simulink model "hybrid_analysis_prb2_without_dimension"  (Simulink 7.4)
settings: Solver=ode4  SolverMode=SingleTasking  StartTime=0.0  StopTime=60.0  FixedStep=0.0005  RelTol=1e-3
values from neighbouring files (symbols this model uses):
  AR1 = 1    [prb2.m]
  AR2 = 4.125    [prb2.m]
  AR3 = 1    [prb2.m]
  c1_mu1 = 1    [prb2.m]
  c1_mu2 = 1    [prb2.m]
  c2_mu1 = 0.1316    [prb2.m]
  c2_mu2 = 0.0001748    [prb2.m]
  c3_mu1 = 1    [prb2.m]
  c3_mu2 = 1    [prb2.m]
  Hf = 0.310    (= 0.31)    [prb2.m]
  Ici = 0.009020    (= 0.00902)    [prb2.m]
  Ici12 = It2 - It    (= 0.0149238079833)    [prb2.m]
  Icr = 0.005806    [prb2.m]
  Icr12 = Icr + Isi/(R1*R1) + Ici/(R2*R2)    (= 0.0366753653)    [prb2.m]
  Isi = 0.001020    (= 0.00102)    [prb2.m]
  Isi12 = It1 - It    (= 0.00429856082609)    [prb2.m]
  Isr = 1    [prb2.m]
  It = 0.05623    [prb2.m]
  It1 = It + Isi + R1*R1*Icr + R1*R1*Ici/(R2*R2)    (= 0.0605285608261)    [prb2.m]
  It2 = It + Ici + R2*R2*Icr + R2*R2*Isi/(R1*R1)    (= 0.0711538079833)    [prb2.m]
  Iwf = 2.8    [prb2.m]
  Ks = 6742.0    (= 6742)    [prb2.m]
  M = 1644.0 + 125.0    (= 1769)    [prb2.m]
  m_s_to_km_h = 3.6    [prb2.m]
  Pc1init = 0    [prb2.m]
  Pc1max = 1    [prb2.m]
  Pc2init = 0    [prb2.m]
  Pc2max = 400.0    (= 400)    [prb2.m]
  Pc3init = 0    [prb2.m]
  Pc3max = 1    [prb2.m]
  pres_index = [-5,5]    [prb2.m]
  R1 = Rci*Rsi/(1-Rci*Rcr)    (= 0.342353138929)    [prb2.m]
  R2 = Rci    (= 0.6379)    [prb2.m]
  R4 = 1    [prb2.m]
  Rci = 0.6379    [prb2.m]
  Rcr = 0.7045    [prb2.m]
  Rd = 0.3521    [prb2.m]
  Rr = 1    [prb2.m]
  Rsi = 0.2955    [prb2.m]
  Rsr = 1    [prb2.m]
  tau1off = 0    [prb2.m]
  tau1on = 1    [prb2.m]
  tau2off = 0    [prb2.m]
  tau2on = 1    [prb2.m]
  tau3off = 0    [prb2.m]
  tau3on = 1    [prb2.m]
  Ts_init = 0    [prb2.m]
  V_init = 0    [prb2.m]
  Wt_init = 0    [prb2.m]
undefined symbols (not defined in the file or in its folder): c1_table, c2_table, c3_table, shift_1_2, shift_2_1, trans, trans_v1_1
libraries: simulink x1
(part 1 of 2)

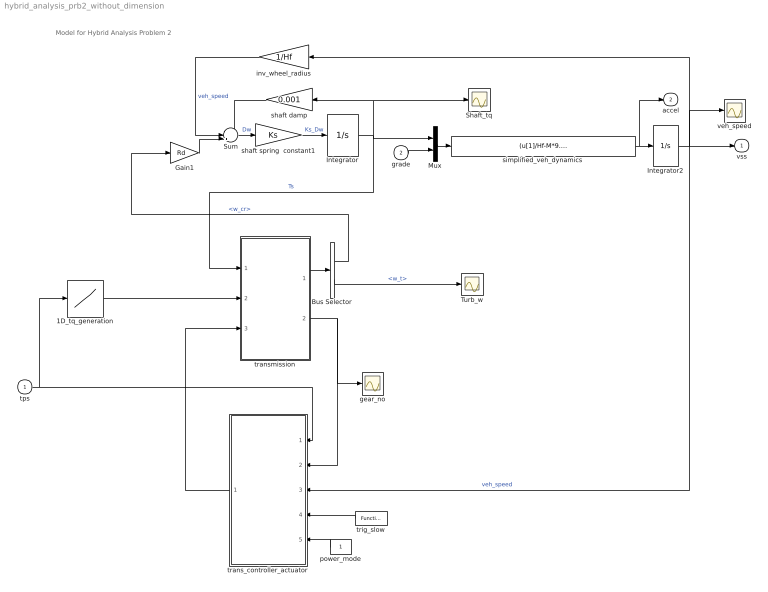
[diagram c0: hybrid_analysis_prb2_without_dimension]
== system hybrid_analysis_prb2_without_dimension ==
  note: Model for Hybrid Analysis Problem 2
  tps : Inport  Description=|
      | begin dimension       
      | output _ : [(scalar)];
      | end dimension
  grade : Inport  Description=|  Port=2
      | begin dimension               
      | output _ : [(angle radian 1)];
      | end dimension
  1D_tq_generation : Lookup  Description=|  InputValues=[0 100]  Table=[30 200]
      | begin dimension                                                
      | input 1 : [(scalar)];                                          
      | output 1 : [(length metre 2, mass kilogram 1, time second -2)];
      | end dimension
  Bus Selector : BusSelector  OutputSignals=w_cr,w_t
  Gain1 : Gain  Gain=Rd
  Integrator : Integrator  InitialCondition=Ts_init
  Integrator2 : Integrator  InitialCondition=V_init
  Mux : Mux  Inputs=2
  Shaft_tq : Scope
  Sum : Sum  Inputs=--+
  Turb_w : Scope
  gear_no : Scope
  inv_wheel_radius : Gain  Description=|  Gain=1/Hf
      | begin dimension                  
      | constant 1 : [(length metre -1)];
      | end dimension
  power_mode : Constant  Description=|
      | begin dimension       
      | output _ : [(scalar)];
      | end dimension
  shaft damp : Gain  Gain=0.001
  shaft spring  constant1 : Gain  Gain=Ks
  simplified_veh_dynamics : Fcn  Expr=(u[1]/Hf-M*9.81*sin(u[2]))/(M+2*Iwf/(Hf*Hf))
  trans_controller_actuator : Subsystem  AncestorBlock=trans/trans_v1_1
  transmission : Subsystem
  trig_slow : simulink/Ports & Subsystems/Function-Call Generator  sample_time=.001  numberOfIterations=1
  veh_speed : Scope
  vss : Outport  Description=|
      | begin dimension                              
      | input _ : [(length metre 1, time second -1)];
      | end dimension
  accel : Outport  Description=|  Port=2
      | begin dimension                              
      | input _ : [(length metre 1, time second -2)];
      | end dimension
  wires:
  transmission/2(current_gear) -> trans_controller_actuator/2(a_gear), gear_no/1
  power_mode/1 -> trans_controller_actuator/5(p_e_switch)
  simplified_veh_dynamics/1 -> Integrator2/1, accel/1
  Mux/1 -> simplified_veh_dynamics/1
  Integrator2/1 -> trans_controller_actuator/3(vss), vss/1, veh_speed/1, inv_wheel_radius/1  "veh_speed"
  grade/1 -> Mux/2
  transmission/1(omegas) -> Bus Selector/1
  tps/1 -> trans_controller_actuator/1(tps), 1D_tq_generation/1
  Integrator/1 -> Mux/1, Shaft_tq/1, shaft damp/1, transmission/1(T_s)  "Ts"
  trig_slow/1 -> trans_controller_actuator/4(trig_trans_slow)
  Sum/1 -> shaft spring  constant1/1  "Dw"
  shaft spring  constant1/1 -> Integrator/1  "Ks_Dw"
  Bus Selector/1 -> Gain1/1  "<w_cr>"
  inv_wheel_radius/1 -> Sum/2  "veh_speed"
  1D_tq_generation/1 -> transmission/2(T_t)
  trans_controller_actuator/1(pcs) -> transmission/3(pc)
  Gain1/1 -> Sum/3
  shaft damp/1 -> Sum/1
  Bus Selector/2 -> Turb_w/1  "<w_t>"

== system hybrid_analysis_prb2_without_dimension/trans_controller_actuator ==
  note: "Execution Context Diagram" At this level, 1 Simulink Subsystem per execution context (e.g. background, pip, cid, 1ms, 2ms, 4ms, etc.) is required. There are no C-specs at this level.
  tps : Inport
  a_gear : Inport  Port=2
  vss : Inport  Port=3
  trig_trans_slow : Inport  Port=4
  p_e_switch : Inport  Port=5
  IC : InitialCondition  Value=Pc1init
  IC1 : InitialCondition  Value=Pc2init
  IC2 : InitialCondition  Value=Pc3init
  Mux6 : Mux  Inputs=3
  Mux7 : Mux  Inputs=3
  clutch_actuators : Subsystem
  trans_slow : Subsystem
  pcs : Outport  InitialOutput=0
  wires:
  a_gear/1 -> trans_slow/5(a_gear)
  p_e_switch/1 -> trans_slow/4(p_e_switch)
  vss/1 -> trans_slow/3(vss)
  tps/1 -> trans_slow/2(tps)
  trig_trans_slow/1 -> trans_slow/1(trig_trans_slow)
  trans_slow/1(Pc1) -> IC/1
  trans_slow/2(Pc2) -> IC1/1
  IC/1 -> Mux7/1  "pc1"
  IC2/1 -> Mux7/3  "pc3"
  IC1/1 -> Mux7/2  "pc2"
  clutch_actuators/1(pc1) -> Mux6/1
  clutch_actuators/2(pc2) -> Mux6/2
  clutch_actuators/3(pc3) -> Mux6/3
  Mux6/1 -> pcs/1
  Mux7/1 -> clutch_actuators/1(pcs)
  trans_slow/3(Pc3) -> IC2/1

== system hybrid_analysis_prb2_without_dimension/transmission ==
  note: References: - Kim, J. and Cho, D., "An Automatic Transmission Model for Vehicle Control," Proc. IEEE Conf. on ITS, Nov. 1997, pp. 759-764. - D. Cho and J.K. Hedrick: "Automotive Powertrain Modeling for Control", ASME Trans. V111, Dec. 1989, pp. 568-576. - Butts, K., "Analysis Needs for Automotive Powertrain Control," Proceedings of The 7th Mechatronics Forum International Conference, September 6-8 2000, Atlanta, Georgia.
  T_s : Inport  Description=|
      | begin dimension                                                
      | output _ : [(length metre 2, mass kilogram 1, time second -2)];
      | end dimension
  T_t : Inport  Description=|  Port=2
      | begin dimension                                                
      | output _ : [(length metre 2, mass kilogram 1, time second -2)];
      | end dimension
  pc : Inport  Description=|  Port=3
      | begin dimension                                                 
      | output _ : [(length metre -1, mass kilogram 1, time second -2)];
      | end dimension
  Memory : Memory  X0=1
  Memory1 : Memory  X0=1
  compute_states : Subsystem
  pressure_to_torque : Subsystem
  reaction_torques : Subsystem
  omegas : Outport  Description=|
      | begin dimension                               
      | output _ : [(angle radian 1, time second -1)];
      | end dimension
  current_gear : Outport  Description=|  Port=2
      | begin dimension      
      | input _ : [(scalar)];
      | end dimension
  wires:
  pc/1 -> pressure_to_torque/1(pcs)
  T_t/1 -> reaction_torques/2(T_t), compute_states/2(T_t)
  T_s/1 -> reaction_torques/1(T_s), compute_states/1(T_s)
  pressure_to_torque/1(T_c) -> reaction_torques/3(T_c), compute_states/3(T_c)
  compute_states/3(gear) -> current_gear/1, Memory/1
  compute_states/1(states) -> omegas/1
  compute_states/2(derivatives) -> Memory1/1
  Memory1/1 -> reaction_torques/4(omega_dots)
  Memory/1 -> reaction_torques/5(current_gear)
  reaction_torques/1(RTs) -> compute_states/4(RTs)

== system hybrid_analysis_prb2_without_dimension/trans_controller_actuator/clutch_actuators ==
  note: This models the application of hydraulic pressure to the clutches and bands as first order lags Pc/Pc_max = 1/(tau*s +1) where each clutch has a distinct tau_on and tau_off.
  pcs : Inport
  Demux : Demux  Outputs=3
  Integrator : Integrator  InitialCondition=[Pc1init,Pc2init,Pc3init]
  Mux3 : Mux  Inputs=3
  Product2 : Product  Inputs=*/
  Sum3 : Sum  Inputs=-+|
  check_pc1 : Subsystem
  check_pc2 : Subsystem
  check_pc3 : Subsystem
  clutch_time_constant : Subsystem
  pc1 : Outport
  pc2 : Outport  Port=2
  pc3 : Outport  Port=3
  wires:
  Product2/1 -> Integrator/1
  Integrator/1 -> Demux/1, Sum3/1
  clutch_time_constant/3(tau3) -> Mux3/3
  clutch_time_constant/2(tau2) -> Mux3/2
  clutch_time_constant/1(tau1) -> Mux3/1
  Mux3/1 -> Product2/2
  pcs/1 -> Sum3/2, clutch_time_constant/1(pcs)
  Sum3/1 -> Product2/1
  check_pc1/1(pc1) -> pc1/1
  check_pc2/1(pc2) -> pc2/1
  check_pc3/1(pc3) -> pc3/1
  Demux/2 -> check_pc2/1(pcs)  "pc2"
  Demux/1 -> check_pc1/1(pcs)  "pc1"
  Demux/3 -> check_pc3/1(pcs)  "pc3"

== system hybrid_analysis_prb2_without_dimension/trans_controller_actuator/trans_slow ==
  note: Note: The controller should control clutch pressures and not torques. This will be fixed in the next release.
  trig_trans_slow : Inport
  tps : Inport  Port=2
  vss : Inport  Port=3
  p_e_switch : Inport  Port=4
  a_gear : Inport  Port=5
  trans_slow_ctl : Stateflow chart  TreatAsAtomicUnit=on
  trans_slow_torques : Subsystem  TreatAsAtomicUnit=on
  Pc1 : Outport  InitialOutput=0
  Pc2 : Outport  Port=2  InitialOutput=0
  Pc3 : Outport  Port=3  InitialOutput=0
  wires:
  trans_slow_torques/3(Pc3) -> Pc3/1
  trans_slow_torques/2(Pc2) -> Pc2/1
  trans_slow_torques/1(Pc1) -> Pc1/1
  trans_slow_ctl/1(do_trans_slow_torques) -> trans_slow_torques/Trigger  "do_trans_slow_torques"
  trig_trans_slow/1 -> trans_slow_ctl/Trigger
  a_gear/1 -> trans_slow_torques/4(a_gear)
  p_e_switch/1 -> trans_slow_torques/3(p_e_switch)
  vss/1 -> trans_slow_torques/2(vss)
  tps/1 -> trans_slow_torques/1(tps)

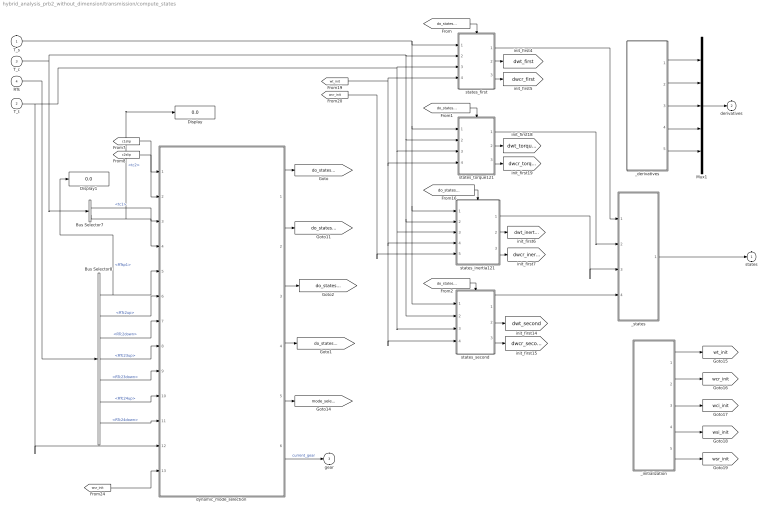
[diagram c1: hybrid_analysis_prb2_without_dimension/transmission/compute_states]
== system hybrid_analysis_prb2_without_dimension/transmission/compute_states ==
  T_s : Inport
  T_t : Inport  Port=2
  T_c : Inport  Port=3
  RTs : Inport  Port=4
  Bus Selector7 : BusSelector  OutputSignals=tc1,tc2
  Bus Selector8 : BusSelector  OutputSignals=RTsp1,RTc2up,RTc2down,RTc23up,RTc23down,RTc24up,RTc24down
  Display : Display
  Display1 : Display
  Mux1 : Mux  Inputs=5
  _derivatives : Subsystem  Description=Merge
  _initialization : Subsystem  Description=Merge
  _states : Subsystem  Description=Merge
  dynamic_mode_selection : Stateflow chart
  states_first : Subsystem  TreatAsAtomicUnit=on
  states_inertia121 : Subsystem  TreatAsAtomicUnit=on
  states_second : Subsystem  TreatAsAtomicUnit=on
  states_torque121 : Subsystem  TreatAsAtomicUnit=on
  states : Outport
  derivatives : Outport  Port=2
  gear : Outport  Port=3
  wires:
  [do_states_second] -> states_second/Enable
  [do_states_inertia121] -> states_inertia121/Enable
  [do_states_torque121] -> states_torque121/Enable
  [c2slip] -> dynamic_mode_selection/2(c2slip)
  [c1slip] -> dynamic_mode_selection/1(c1slip)
  Bus Selector7/1 -> dynamic_mode_selection/3(Tc1)  "<tc1>"
  T_c/1 -> Bus Selector7/1, states_first/2(T_c), states_torque121/2(T_c), states_inertia121/2(T_c), states_second/2(T_c)
  T_t/1 -> dynamic_mode_selection/12(Tt), states_first/3(T_t), states_torque121/3(T_t), states_inertia121/3(T_t), states_second/3(T_t)
  [do_states_first] -> states_first/Enable
  T_s/1 -> states_first/1(T_s), states_torque121/1(T_s), states_inertia121/1(T_s), states_second/1(T_s)
  states_first/1(states) -> _states/1(omegas)
  states_torque121/1(states) -> _states/2(omegas1)
  states_inertia121/1(states) -> _states/3(omegas2)
  states_second/1(states) -> _states/4(omegas3)
  [wt_init] -> states_first/4(wt_init), states_torque121/4(wt_init), states_inertia121/4(wt_init), states_second/4(wt_init1)
  [wcr_init] -> states_inertia121/5(wcr_init)
  states_first/2(wt_dot) -> [dwt_first]
  states_first/3(wcr_dot) -> [dwcr_first]
  states_torque121/2(wt_dot) -> [dwt_torque121]
  states_torque121/3(wcr_dot) -> [dwcr_torque121]
  states_inertia121/2(wt_dot) -> [dwt_inertia121]
  states_inertia121/3(wcr_dot) -> [dwcr_inertia121]
  states_second/2(wt_dot) -> [dwt_second]
  states_second/3(wcr_dot) -> [dwcr_second]
  _initialization/5(wsr_init) -> [wsr_init]
  _initialization/4(wsi_init) -> [wsi_init]
  _states/1(reaction_torques) -> states/1
  _derivatives/1(wt_dot) -> Mux1/1
  _derivatives/2(wcr_dot) -> Mux1/2
  _derivatives/3(wci_dot) -> Mux1/3
  _derivatives/4(wsi_dot) -> Mux1/4
  _derivatives/5(wsr_dot) -> Mux1/5
  Mux1/1 -> derivatives/1
  _initialization/1(wt_init) -> [wt_init]
  _initialization/3(wci_init) -> [wci_init]
  _initialization/2(wcr_init) -> [wcr_init]
  Bus Selector7/2 -> dynamic_mode_selection/4(Tc2), Display/1  "<tc2>"
  dynamic_mode_selection/6(a_gear) -> gear/1  "current_gear"
  dynamic_mode_selection/4(second) -> [do_states_second]
  dynamic_mode_selection/1(first) -> [do_states_first]
  dynamic_mode_selection/5(mode_select) -> [mode_select]
  Bus Selector8/1 -> dynamic_mode_selection/5(RTsp1), Display1/1  "<RTsp1>"
  RTs/1 -> Bus Selector8/1
  Bus Selector8/3 -> dynamic_mode_selection/7(RTc2down)  "<RTc2down>"
  Bus Selector8/4 -> dynamic_mode_selection/8(RTc23up)  "<RTc23up>"
  Bus Selector8/5 -> dynamic_mode_selection/9(RTc23down)  "<RTc23down>"
  Bus Selector8/6 -> dynamic_mode_selection/10(RTc24up)  "<RTc24up>"
  Bus Selector8/7 -> dynamic_mode_selection/11(RTc24down)  "<RTc24down>"
  Bus Selector8/2 -> dynamic_mode_selection/6(RTc2up)  "<RTc2up>"
  [wsr_init] -> dynamic_mode_selection/13(w_sr)
  dynamic_mode_selection/2(torque121) -> [do_states_torque121]
  dynamic_mode_selection/3(inertia121) -> [do_states_inertia121]

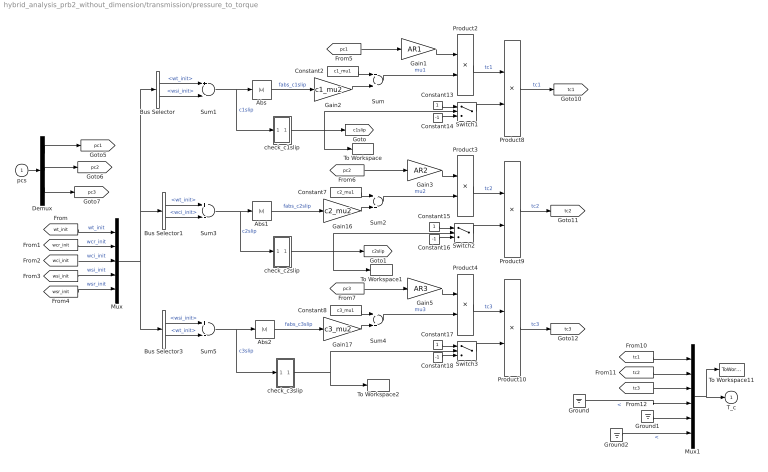
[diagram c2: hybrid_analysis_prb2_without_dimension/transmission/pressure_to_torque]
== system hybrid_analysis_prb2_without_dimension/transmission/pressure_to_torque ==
  pcs : Inport
  Abs : Abs
  Abs1 : Abs
  Abs2 : Abs
  Bus Selector : BusSelector  OutputSignals=wt_init,wsi_init
  Bus Selector1 : BusSelector  OutputSignals=wt_init,wci_init
  Bus Selector3 : BusSelector  OutputSignals=wsi_init,wt_init
  Constant13 : Constant
  Constant14 : Constant  Value=-1
  Constant15 : Constant
  Constant16 : Constant  Value=-1
  Constant17 : Constant
  Constant18 : Constant  Value=-1
  Constant2 : Constant  Value=c1_mu1
  Constant7 : Constant  Value=c2_mu1
  Constant8 : Constant  Value=c3_mu1
  Demux : Demux  Outputs=3
  Gain1 : Gain  Gain=AR1
  Gain16 : Gain  Gain=c2_mu2
  Gain17 : Gain  Gain=c3_mu2
  Gain2 : Gain  Gain=c1_mu2
  Gain3 : Gain  Gain=AR2
  Gain5 : Gain  Gain=AR3
  Ground : Ground
  Ground1 : Ground
  Ground2 : Ground
  Mux : Mux  Inputs=5
  Mux1 : Mux  Inputs=6
  Product{2..4,8..10} (6 alike) : Product
  Sum : Sum  Inputs=2
  Sum1 : Sum  Inputs=+-
  Sum2 : Sum  Inputs=2
  Sum3 : Sum  Inputs=+-
  Sum4 : Sum  Inputs=2
  Sum5 : Sum  Inputs=+-
  Switch1 : Switch
  Switch2 : Switch
  Switch3 : Switch
  To Workspace : ToWorkspace  VariableName=c1slip  SampleTime=-1  SaveFormat=Array
  To Workspace1 : ToWorkspace  VariableName=c2slip  SampleTime=-1  SaveFormat=Array
  To Workspace11 : ToWorkspace  VariableName=tc  SaveFormat=Array
  To Workspace2 : ToWorkspace  VariableName=c3slip  SampleTime=-1  SaveFormat=Array
  check_c1slip : Subsystem
  check_c2slip : Subsystem
  check_c3slip : Subsystem
  T_c : Outport
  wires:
  Gain1/1 -> Product2/1
  [pc1] -> Gain1/1
  Sum/1 -> Product2/2  "mu1"
  Bus Selector/2 -> Sum1/2  "<wsi_init>"
  Bus Selector/1 -> Sum1/1  "<wt_init>"
  Abs/1 -> Gain2/1  "fabs_c1slip"
  Sum1/1 -> Abs/1, check_c1slip/1(In1)  "c1slip"
  Constant2/1 -> Sum/1
  Gain2/1 -> Sum/2
  Product2/1 -> Product8/1  "tc1"
  check_c1slip/1(Out1) -> [c1slip], Switch1/2, To Workspace/1
  Switch1/1 -> Product8/2
  Constant13/1 -> Switch1/1
  Constant14/1 -> Switch1/3
  Gain3/1 -> Product3/1
  Sum2/1 -> Product3/2  "mu2"
  Bus Selector1/1 -> Sum3/1  "<wt_init>"
  Bus Selector1/2 -> Sum3/2  "<wci_init>"
  Gain16/1 -> Sum2/2
  Abs1/1 -> Gain16/1  "fabs_c2slip"
  Sum3/1 -> Abs1/1, check_c2slip/1(In1)  "c2slip"
  [pc2] -> Gain3/1
  Constant7/1 -> Sum2/1
  [pc3] -> Gain5/1
  Gain5/1 -> Product4/1
  Product3/1 -> Product9/1  "tc2"
  Switch2/1 -> Product9/2
  Constant15/1 -> Switch2/1
  Constant16/1 -> Switch2/3
  check_c2slip/1(Out1) -> [c2slip], Switch2/2, To Workspace1/1
  [wt_init] -> Mux/1  "wt_init"
  [wcr_init] -> Mux/2  "wcr_init"
  [wsi_init] -> Mux/4  "wsi_init"
  [wsr_init] -> Mux/5  "wsr_init"
  [wci_init] -> Mux/3  "wci_init"
  Bus Selector3/1 -> Sum5/1  "<wsi_init>"
  Bus Selector3/2 -> Sum5/2  "<wt_init>"
  Abs2/1 -> Gain17/1  "fabs_c3slip"
  Sum5/1 -> Abs2/1, check_c3slip/1(In1)  "c3slip"
  Gain17/1 -> Sum4/2
  Constant8/1 -> Sum4/1
  Sum4/1 -> Product4/2  "mu3"
  check_c3slip/1(Out1) -> To Workspace2/1, Switch3/2
  Product4/1 -> Product10/1  "tc3"
  Switch3/1 -> Product10/2
  Constant17/1 -> Switch3/1
  Constant18/1 -> Switch3/3
  [tc1] -> Mux1/1
  [tc2] -> Mux1/2
  Ground/1 -> Mux1/4  "<"
  Ground1/1 -> Mux1/5
  [tc3] -> Mux1/3
  Ground2/1 -> Mux1/6  "<"
  Demux/1 -> [pc1]
  Demux/2 -> [pc2]
  Demux/3 -> [pc3]
  pcs/1 -> Demux/1
  Mux1/1 -> To Workspace11/1, T_c/1
  Product9/1 -> [tc2]  "tc2"
  Product10/1 -> [tc3]  "tc3"
  Product8/1 -> [tc1]  "tc1"
  Mux/1 -> Bus Selector/1, Bus Selector1/1, Bus Selector3/1

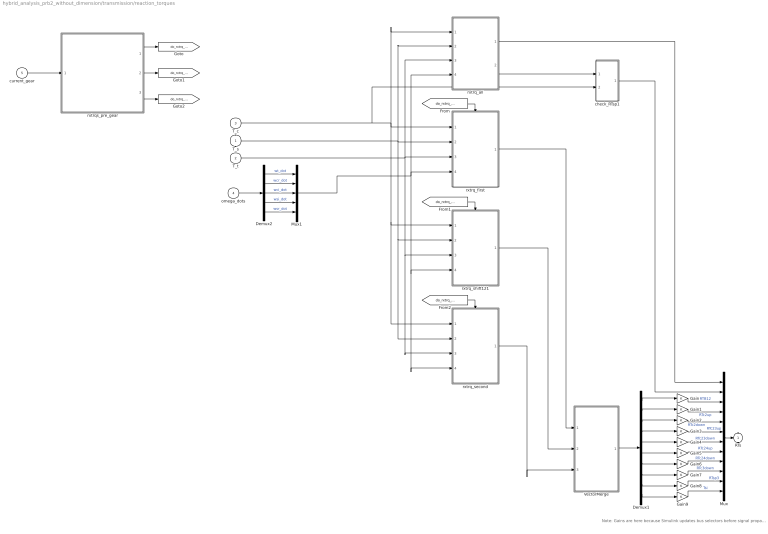
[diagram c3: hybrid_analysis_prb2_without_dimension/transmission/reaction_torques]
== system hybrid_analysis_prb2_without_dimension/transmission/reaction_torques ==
  note: Note: Gains are here because Simulink updates bus selectors before signal propagation. This seems to cause errors here -- temporary solution.
  T_s : Inport
  T_t : Inport  Port=2
  T_c : Inport  Port=3
  omega_dots : Inport  Port=4
  current_gear : Inport  Port=5
  Demux1 : Demux  Outputs=10
  Demux2 : Demux  Outputs=5
  Gain{,1..9} (10 alike) : Gain
  Mux : Mux  Inputs=12
  Mux1 : Mux  Inputs=5
  VectorMerge : Subsystem
  check_RTsp1 : Subsystem
  rxtrq_all : Subsystem
  rxtrq_first : Subsystem  TreatAsAtomicUnit=on
  rxtrq_second : Subsystem  TreatAsAtomicUnit=on
  rxtrq_shift121 : Subsystem  TreatAsAtomicUnit=on
  rxtrqs_pre_gear : Stateflow chart
  RTs : Outport  InitialOutput=[0,0,0,0,0,0,0,0,0,0]
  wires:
  current_gear/1 -> rxtrqs_pre_gear/1(gear)
  rxtrqs_pre_gear/1(do_rxtrq_first) -> [do_rxtrq_first]
  rxtrqs_pre_gear/2(do_rxtrq_shift121) -> [do_rxtrq_shift121]
  rxtrqs_pre_gear/3(do_rxtrq_second) -> [do_rxtrq_second]
  T_t/1 -> rxtrq_first/3(T_t), rxtrq_all/3(T_t), rxtrq_shift121/3(T_t), rxtrq_second/3(T_t)
  T_s/1 -> rxtrq_first/2(T_s), rxtrq_all/2(T_s), rxtrq_shift121/2(T_s), rxtrq_second/2(T_s)
  [do_rxtrq_first] -> rxtrq_first/Enable
  [do_rxtrq_shift121] -> rxtrq_shift121/Enable
  [do_rxtrq_second] -> rxtrq_second/Enable
  rxtrq_all/2(RTsp1) -> check_RTsp1/1(In1)
  rxtrq_second/1(reaction_torques) -> VectorMerge/3(omegas2)
  rxtrq_shift121/1(reaction_torques) -> VectorMerge/2(omegas1)
  rxtrq_first/1(reaction_torques) -> VectorMerge/1(omegas)
  VectorMerge/1(reaction_torques) -> Demux1/1
  rxtrq_all/1(RTc1up) -> Mux/1
  check_RTsp1/1(Out1) -> Mux/2
  Demux1/10 -> Gain9/1
  Gain9/1 -> Mux/12  "Tsi"
  Demux1/9 -> Gain8/1
  Gain8/1 -> Mux/11  "RTsp3"
  Demux1/8 -> Gain7/1
  Gain7/1 -> Mux/10  "RTc3down"
  Demux1/7 -> Gain6/1
  Gain6/1 -> Mux/9  "RTc24down"
  Demux1/6 -> Gain5/1
  Gain5/1 -> Mux/8  "RTc24up"
  Demux1/5 -> Gain4/1
  Gain4/1 -> Mux/7  "RTc23down"
  Demux1/4 -> Gain3/1
  Gain3/1 -> Mux/6  "RTc23up"
  Demux1/3 -> Gain2/1
  Gain2/1 -> Mux/5  "RTc2down"
  Demux1/2 -> Gain1/1
  Gain1/1 -> Mux/4  "RTc2up"
  Demux1/1 -> Gain/1
  Gain/1 -> Mux/3  "RTB12"
  T_c/1 -> rxtrq_first/1(T_c), rxtrq_all/1(T_c), rxtrq_shift121/1(T_c), rxtrq_second/1(T_c), check_RTsp1/2(In2)
  Demux2/1 -> Mux1/1  "wt_dot"
  Demux2/5 -> Mux1/5  "wsr_dot"
  Demux2/2 -> Mux1/2  "wcr_dot"
  Demux2/3 -> Mux1/3  "wci_dot"
  Demux2/4 -> Mux1/4  "wsi_dot"
  omega_dots/1 -> Demux2/1
  Mux1/1 -> rxtrq_first/4(omega_dots), rxtrq_all/4(omega_dots), rxtrq_shift121/4(omega_dots), rxtrq_second/4(omega_dots)
  Mux/1 -> RTs/1

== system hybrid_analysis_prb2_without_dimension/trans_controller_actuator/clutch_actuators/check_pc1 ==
  pcs : Inport
  Constant : Constant  Value=1.0
  Constant1 : Constant  Value=0
  Constant2 : Constant  Value=Pc1max
  Constant3 : Constant  Value=1.0
  Constant4 : Constant  Value=Pc1max
  Relational Operator : RelationalOperator  Operator=<
  Relational Operator1 : RelationalOperator  Operator=<=
  Sum7 : Sum  Inputs=+-
  Switch : Switch  Threshold=0.5
  Switch1 : Switch  Threshold=0.5
  pc1 : Outport
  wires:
  Constant/1 -> Relational Operator/2
  Relational Operator/1 -> Switch/2
  Constant1/1 -> Switch/1
  pcs/1 -> Relational Operator/1, Switch/3
  Constant2/1 -> Sum7/1
  Sum7/1 -> Relational Operator1/1
  Constant3/1 -> Relational Operator1/2
  Relational Operator1/1 -> Switch1/2
  Constant4/1 -> Switch1/1
  Switch/1 -> Sum7/2, Switch1/3  "pc1"
  Switch1/1 -> pc1/1  "pc1"

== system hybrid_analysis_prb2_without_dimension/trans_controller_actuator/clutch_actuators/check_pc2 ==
  pcs : Inport
  Constant : Constant  Value=1.0
  Constant1 : Constant  Value=0
  Constant2 : Constant  Value=Pc2max
  Constant3 : Constant  Value=1.0
  Constant4 : Constant  Value=Pc2max
  Relational Operator : RelationalOperator  Operator=<
  Relational Operator1 : RelationalOperator  Operator=<=
  Sum7 : Sum  Inputs=+-
  Switch : Switch  Threshold=0.5
  Switch1 : Switch  Threshold=0.5
  pc2 : Outport
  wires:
  Switch1/1 -> pc2/1  "pc2"
  Switch/1 -> Switch1/3, Sum7/2  "pc2"
  Constant4/1 -> Switch1/1
  Relational Operator1/1 -> Switch1/2
  Constant3/1 -> Relational Operator1/2
  Sum7/1 -> Relational Operator1/1
  Constant2/1 -> Sum7/1
  pcs/1 -> Switch/3, Relational Operator/1
  Constant1/1 -> Switch/1
  Relational Operator/1 -> Switch/2
  Constant/1 -> Relational Operator/2

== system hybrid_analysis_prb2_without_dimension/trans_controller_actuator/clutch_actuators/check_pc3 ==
  pcs : Inport
  Constant : Constant  Value=1.0
  Constant1 : Constant  Value=0
  Constant2 : Constant  Value=Pc3max
  Constant3 : Constant  Value=1.0
  Constant4 : Constant  Value=Pc3max
  Relational Operator : RelationalOperator  Operator=<
  Relational Operator1 : RelationalOperator  Operator=<=
  Sum7 : Sum  Inputs=+-
  Switch : Switch  Threshold=0.5
  Switch1 : Switch  Threshold=0.5
  pc3 : Outport
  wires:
  Constant/1 -> Relational Operator/2
  Relational Operator/1 -> Switch/2
  Constant1/1 -> Switch/1
  pcs/1 -> Relational Operator/1, Switch/3
  Constant2/1 -> Sum7/1
  Sum7/1 -> Relational Operator1/1
  Constant3/1 -> Relational Operator1/2
  Relational Operator1/1 -> Switch1/2
  Constant4/1 -> Switch1/1
  Switch/1 -> Sum7/2, Switch1/3  "pc3"
  Switch1/1 -> pc3/1  "pc3"

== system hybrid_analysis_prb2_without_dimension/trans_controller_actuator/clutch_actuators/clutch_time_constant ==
  pcs : Inport
  Constant : Constant  Value=tau1on
  Constant1 : Constant  Value=tau1off
  Constant2 : Constant  Value=tau2on
  Constant3 : Constant  Value=tau2off
  Constant4 : Constant  Value=tau3on
  Constant5 : Constant  Value=tau3off
  Demux : Demux  Outputs=3
  Switch1 : Switch  Threshold=1
  Switch2 : Switch  Threshold=1
  Switch3 : Switch  Threshold=1
  tau1 : Outport
  tau2 : Outport  Port=2
  tau3 : Outport  Port=3
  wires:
  pcs/1 -> Demux/1
  Constant/1 -> Switch1/1
  Constant1/1 -> Switch1/3
  Demux/1 -> Switch1/2
  Demux/2 -> Switch2/2
  Constant2/1 -> Switch2/1
  Constant3/1 -> Switch2/3
  Switch2/1 -> tau2/1  "tau2"
  Switch1/1 -> tau1/1  "tau1"
  Demux/3 -> Switch3/2
  Constant4/1 -> Switch3/1
  Constant5/1 -> Switch3/3
  Switch3/1 -> tau3/1  "tau3"

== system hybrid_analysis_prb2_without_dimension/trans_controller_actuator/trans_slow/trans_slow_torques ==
  note: TRANSMISSION CONTROL 1. shift scheduler calculates gear command based on alpha and V 2. clutch pressure controller applies proper pressure to clutches to perform the shift
  tps : Inport
  vss : Inport  Port=2
  p_e_switch : Inport  Port=3
  a_gear : Inport  Port=4
  do_trans_slow_torques : TriggerPort  TriggerType=function-call
  clutch_pressure : Subsystem
  shift_scheduler : Subsystem
  Pc1 : Outport  InitialOutput=0
  Pc2 : Outport  Port=2  InitialOutput=0
  Pc3 : Outport  Port=3  InitialOutput=0
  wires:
  clutch_pressure/3(Pc7) -> Pc3/1
  clutch_pressure/2(Pc6) -> Pc2/1
  clutch_pressure/1(Pc5) -> Pc1/1
  a_gear/1 -> shift_scheduler/4(gear)
  vss/1 -> shift_scheduler/2(vss)
  tps/1 -> shift_scheduler/1(tps)
  p_e_switch/1 -> shift_scheduler/3(p_e_switch)
  shift_scheduler/1(ngear) -> clutch_pressure/1(ngear1)

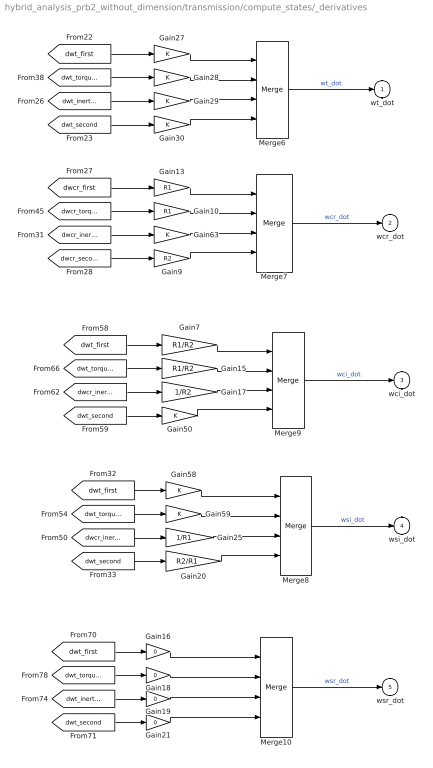
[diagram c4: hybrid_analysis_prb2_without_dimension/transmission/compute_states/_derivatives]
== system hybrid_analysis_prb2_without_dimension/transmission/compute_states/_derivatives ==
  Gain10 : Gain  Gain=R1
  Gain13 : Gain  Gain=R1
  Gain15 : Gain  Gain=R1/R2
  Gain{16,18..19,21} (4 alike) : Gain  Gain=0
  Gain17 : Gain  Gain=1/R2
  Gain20 : Gain  Gain=R2/R1
  Gain25 : Gain  Gain=1/R1
  Gain{27..30,50,58..59,63} (8 alike) : Gain
  Gain7 : Gain  Gain=R1/R2
  Gain9 : Gain  Gain=R2
  Merge{6..10} (5 alike) : Merge  Inputs=4
  wt_dot : Outport  InitialOutput=[0,0,0,0,0,0,0,0,0,0]
  wcr_dot : Outport  Port=2  InitialOutput=[0,0,0,0,0,0,0,0,0,0]
  wci_dot : Outport  Port=3  InitialOutput=[0,0,0,0,0,0,0,0,0,0]
  wsi_dot : Outport  Port=4  InitialOutput=[0,0,0,0,0,0,0,0,0,0]
  wsr_dot : Outport  Port=5  InitialOutput=[0,0,0,0,0,0,0,0,0,0]
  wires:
  Merge6/1 -> wt_dot/1  "wt_dot"
  Merge7/1 -> wcr_dot/1  "wcr_dot"
  [dwcr_first] -> Gain13/1
  Gain13/1 -> Merge7/1
  [dwcr_torque121] -> Gain10/1
  Gain10/1 -> Merge7/2
  [dwcr_second] -> Gain9/1
  Gain9/1 -> Merge7/4
  [dwt_first] -> Gain7/1
  Gain7/1 -> Merge9/1
  [dwt_second] -> Gain20/1
  Gain20/1 -> Merge8/4
  Merge8/1 -> wsi_dot/1  "wsi_dot"
  [dwcr_inertia121] -> Gain25/1
  Gain25/1 -> Merge8/3
  [dwt_torque121] -> Gain15/1
  Gain15/1 -> Merge9/2
  [dwcr_inertia121] -> Gain17/1
  Gain17/1 -> Merge9/3
  Merge9/1 -> wci_dot/1  "wci_dot"
  [dwt_first] -> Gain16/1
  Gain16/1 -> Merge10/1
  [dwt_torque121] -> Gain18/1
  Gain18/1 -> Merge10/2
  [dwt_inertia121] -> Gain19/1
  Gain19/1 -> Merge10/3
  [dwt_second] -> Gain21/1
  Gain21/1 -> Merge10/4
  Merge10/1 -> wsr_dot/1  "wsr_dot"
  [dwt_first] -> Gain27/1
  Gain27/1 -> Merge6/1
  [dwt_torque121] -> Gain28/1
  Gain28/1 -> Merge6/2
  [dwt_inertia121] -> Gain29/1
  Gain29/1 -> Merge6/3
  [dwt_second] -> Gain30/1
  Gain30/1 -> Merge6/4
  [dwt_second] -> Gain50/1
  Gain50/1 -> Merge9/4
  [dwt_first] -> Gain58/1
  Gain58/1 -> Merge8/1
  [dwt_torque121] -> Gain59/1
  Gain59/1 -> Merge8/2
  [dwcr_inertia121] -> Gain63/1
  Gain63/1 -> Merge7/3

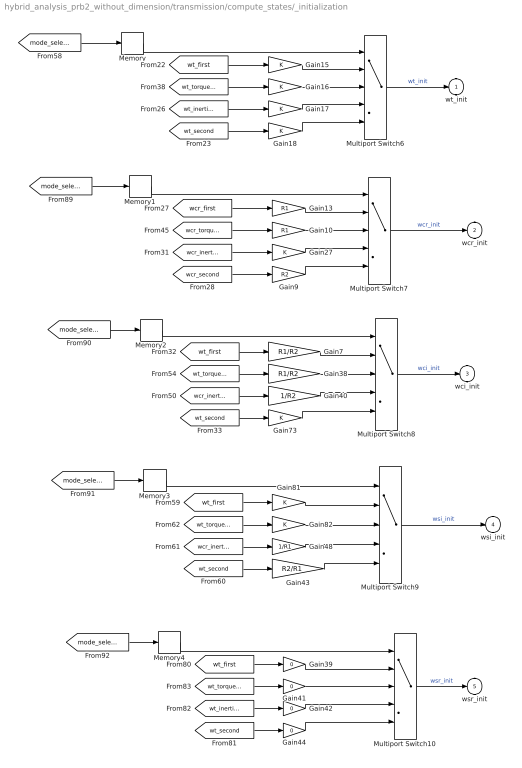
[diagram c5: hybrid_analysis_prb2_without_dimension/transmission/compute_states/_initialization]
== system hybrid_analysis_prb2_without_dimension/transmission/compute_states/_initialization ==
  Gain10 : Gain  Gain=R1
  Gain13 : Gain  Gain=R1
  Gain{15..18,27,73,81..82} (8 alike) : Gain
  Gain38 : Gain  Gain=R1/R2
  Gain{39,41..42,44} (4 alike) : Gain  Gain=0
  Gain40 : Gain  Gain=1/R2
  Gain43 : Gain  Gain=R2/R1
  Gain48 : Gain  Gain=1/R1
  Gain7 : Gain  Gain=R1/R2
  Gain9 : Gain  Gain=R2
  Memory{,1..4} (5 alike) : Memory  X0=1
  Multiport Switch{6..10} (5 alike) : MultiPortSwitch  Inputs=4
  wt_init : Outport  InitialOutput=[0,0,0,0,0,0,0,0,0,0]
  wcr_init : Outport  Port=2  InitialOutput=[0,0,0,0,0,0,0,0,0,0]
  wci_init : Outport  Port=3  InitialOutput=[0,0,0,0,0,0,0,0,0,0]
  wsi_init : Outport  Port=4  InitialOutput=[0,0,0,0,0,0,0,0,0,0]
  wsr_init : Outport  Port=5  InitialOutput=[0,0,0,0,0,0,0,0,0,0]
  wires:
  [wcr_first] -> Gain13/1
  Gain13/1 -> Multiport Switch7/2
  [wcr_torque121] -> Gain10/1
  Gain10/1 -> Multiport Switch7/3
  [wcr_second] -> Gain9/1
  Gain9/1 -> Multiport Switch7/5
  Gain16/1 -> Multiport Switch6/3
  Gain17/1 -> Multiport Switch6/4
  Gain18/1 -> Multiport Switch6/5
  [wcr_inertia121] -> Gain27/1
  Gain27/1 -> Multiport Switch7/4
  Gain15/1 -> Multiport Switch6/2
  [wt_second] -> Gain18/1
  [wt_inertia121] -> Gain17/1
  [wt_torque121] -> Gain16/1
  [wt_first] -> Gain15/1
  Multiport Switch6/1 -> wt_init/1  "wt_init"
  Multiport Switch7/1 -> wcr_init/1  "wcr_init"
  [wt_first] -> Gain7/1
  Gain7/1 -> Multiport Switch8/2
  [wt_torque121] -> Gain38/1
  Gain38/1 -> Multiport Switch8/3
  [wcr_inertia121] -> Gain40/1
  Gain40/1 -> Multiport Switch8/4
  [wt_second] -> Gain73/1
  Gain73/1 -> Multiport Switch8/5
  Memory2/1 -> Multiport Switch8/1
  Multiport Switch8/1 -> wci_init/1  "wci_init"
  Memory3/1 -> Multiport Switch9/1
  Gain43/1 -> Multiport Switch9/5
  Gain48/1 -> Multiport Switch9/4
  Gain81/1 -> Multiport Switch9/2
  Gain82/1 -> Multiport Switch9/3
  [wt_second] -> Gain43/1
  [wcr_inertia121] -> Gain48/1
  [wt_torque121] -> Gain82/1
  [wt_first] -> Gain81/1
  Multiport Switch9/1 -> wsi_init/1  "wsi_init"
  [mode_select] -> Memory3/1
  Gain39/1 -> Multiport Switch10/2
  Gain41/1 -> Multiport Switch10/3
  Gain42/1 -> Multiport Switch10/4
  Gain44/1 -> Multiport Switch10/5
  [wt_first] -> Gain39/1
  [wt_torque121] -> Gain41/1
  [wt_inertia121] -> Gain42/1
  [wt_second] -> Gain44/1
  Memory4/1 -> Multiport Switch10/1
  [mode_select] -> Memory4/1
  Multiport Switch10/1 -> wsr_init/1  "wsr_init"
  [mode_select] -> Memory2/1
  [mode_select] -> Memory1/1
  Memory1/1 -> Multiport Switch7/1
  [mode_select] -> Memory/1
  Memory/1 -> Multiport Switch6/1

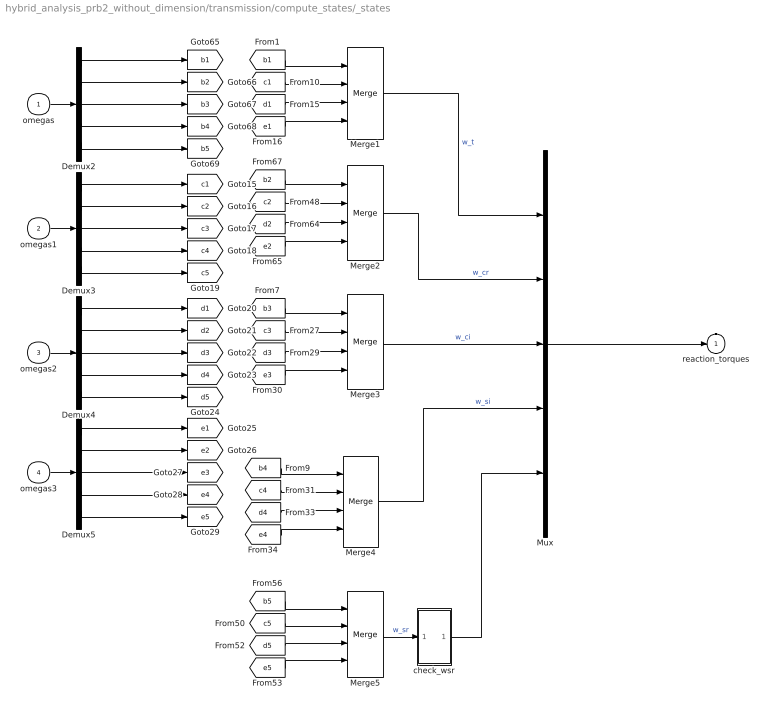
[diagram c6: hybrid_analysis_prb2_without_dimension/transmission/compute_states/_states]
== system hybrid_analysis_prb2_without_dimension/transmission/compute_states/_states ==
  omegas : Inport
  omegas1 : Inport  Port=2
  omegas2 : Inport  Port=3
  omegas3 : Inport  Port=4
  Demux{2..5} (4 alike) : Demux  Outputs=5
  Merge{1..5} (5 alike) : Merge  Inputs=4
  Mux : Mux  Inputs=5
  check_wsr : Subsystem
  reaction_torques : Outport  InitialOutput=[0,0,0,0,0,0,0,0,0,0]
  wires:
  omegas/1 -> Demux2/1
  Demux2/1 -> [b1]
  Demux2/2 -> [b2]
  Demux2/3 -> [b3]
  Demux2/4 -> [b4]
  Demux2/5 -> [b5]
  omegas1/1 -> Demux3/1
  Demux3/1 -> [c1]
  Demux3/2 -> [c2]
  Demux3/3 -> [c3]
  Demux3/4 -> [c4]
  Demux3/5 -> [c5]
  omegas2/1 -> Demux4/1
  Demux4/1 -> [d1]
  Demux4/2 -> [d2]
  Demux4/3 -> [d3]
  Demux4/4 -> [d4]
  Demux4/5 -> [d5]
  omegas3/1 -> Demux5/1
  Demux5/1 -> [e1]
  Demux5/2 -> [e2]
  Demux5/3 -> [e3]
  Demux5/4 -> [e4]
  Demux5/5 -> [e5]
  [b1] -> Merge1/1
  [c1] -> Merge1/2
  [e1] -> Merge1/4
  [d1] -> Merge1/3
  [b2] -> Merge2/1
  [c2] -> Merge2/2
  [e2] -> Merge2/4
  [d2] -> Merge2/3
  [b3] -> Merge3/1
  [c3] -> Merge3/2
  [e3] -> Merge3/4
  [d3] -> Merge3/3
  [b4] -> Merge4/1
  [c4] -> Merge4/2
  [e4] -> Merge4/4
  [d4] -> Merge4/3
  [b5] -> Merge5/1
  [c5] -> Merge5/2
  [e5] -> Merge5/4
  [d5] -> Merge5/3
  Merge3/1 -> Mux/3  "w_ci"
  Merge2/1 -> Mux/2  "w_cr"
  Merge4/1 -> Mux/4  "w_si"
  Merge1/1 -> Mux/1  "w_t"
  Mux/1 -> reaction_torques/1
  Merge5/1 -> check_wsr/1(In1)  "w_sr"
  check_wsr/1(Out1) -> Mux/5

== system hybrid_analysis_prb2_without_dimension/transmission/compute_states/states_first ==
  T_s : Inport
  T_c : Inport  Port=2
  T_t : Inport  Port=3
  wt_init : Inport  Port=4
  Enable : EnablePort  StatesWhenEnabling=reset
  Constant27 : Constant  Value=0
  Gain{7..10} (4 alike) : Gain
  Gain3 : Gain  Gain=R1*Rd
  Gain4 : Gain  Gain=1/It1
  Gain5 : Gain  Gain=R1
  Gain6 : Gain  Gain=R1/R2
  IC : InitialCondition  Value=Wt_init
  Integrator1 : Integrator  InitialConditionSource=external  ShowStatePort=on
  Mux2 : Mux  Inputs=5
  Sum7 : Sum  Inputs=+-
  Terminator : Terminator
  states : Outport
  wt_dot : Outport  Port=2
  wcr_dot : Outport  Port=3
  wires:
  T_s/1 -> Gain3/1
  T_t/1 -> Sum7/1
  Gain3/1 -> Sum7/2
  Sum7/1 -> Gain4/1
  wt_init/1 -> IC/1
  Constant27/1 -> Mux2/5  "wsr"
  Gain5/1 -> Mux2/2  "wcr"
  Gain6/1 -> Mux2/3  "wci"
  Gain7/1 -> Mux2/4  "wsi"
  Gain8/1 -> Mux2/1  "wt"
  Mux2/1 -> states/1
  Integrator1/State -> [wt_first], [wcr_first]
  IC/1 -> Integrator1/2
  Gain4/1 -> Integrator1/1, Gain9/1, Gain10/1  "wt_dot"
  Gain9/1 -> wt_dot/1  "wt_dot"
  Gain10/1 -> wcr_dot/1  "wcr_dot"
  Integrator1/1 -> Gain8/1, Gain5/1, Gain6/1, Gain7/1
  T_c/1 -> Terminator/1

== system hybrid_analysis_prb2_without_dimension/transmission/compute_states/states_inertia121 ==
  note: Note: The wci and wsi calcs are different in some versions of the documentation. These are most likely the correct versions. If spikes occur during shifting, modify the gain on wt->wci to R1/R2 and the gain on wt->wsi to 1.
  T_s : Inport
  T_c : Inport  Port=2
  T_t : Inport  Port=3
  wt_init : Inport  Port=4
  wcr_init : Inport  Port=5
  Enable : EnablePort  StatesWhenEnabling=reset
  Bus Selector3 : BusSelector  OutputSignals=tc2
  Constant26 : Constant  Value=0
  Gain11 : Gain  Gain=1/R2
  Gain12 : Gain  Gain=1/R1
  Gain14 : Gain  Gain=1/R2
  Gain15 : Gain  Gain=Rd
  Gain16 : Gain
  Gain17 : Gain
  Gain4 : Gain  Gain=1/It
  Gain5 : Gain  Gain=1/Icr12
  Integrator2 : Integrator  InitialConditionSource=external  ShowStatePort=on
  Integrator3 : Integrator  InitialConditionSource=external  ShowStatePort=on
  Mux : Mux  Inputs=5
  Sum7 : Sum  Inputs=+-
  Sum8 : Sum  Inputs=+-
  states : Outport
  wt_dot : Outport  Port=2
  wcr_dot : Outport  Port=3
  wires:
  Sum7/1 -> Gain4/1
  T_t/1 -> Sum7/1
  T_c/1 -> Bus Selector3/1
  Bus Selector3/1 -> Sum7/2, Gain14/1  "<tc2>"
  wt_init/1 -> Integrator3/2
  Integrator3/State -> [wt_inertia121]
  Gain16/1 -> Mux/1  "wt"
  Gain14/1 -> Sum8/1
  Gain15/1 -> Sum8/2
  T_s/1 -> Gain15/1
  Sum8/1 -> Gain5/1
  wcr_init/1 -> Integrator2/2
  Integrator2/State -> [wcr_inertia121]
  Gain4/1 -> Integrator3/1, wt_dot/1  "wt_dot"
  Gain5/1 -> Integrator2/1, wcr_dot/1  "wcr_dot"
  Gain12/1 -> Mux/4  "wsi"
  Gain11/1 -> Mux/3  "wci"
  Constant26/1 -> Mux/5  "wsr"
  Mux/1 -> states/1
  Integrator3/1 -> Gain16/1
  Integrator2/1 -> Gain11/1, Gain17/1, Gain12/1  "wcr"
  Gain17/1 -> Mux/2  "wcr"

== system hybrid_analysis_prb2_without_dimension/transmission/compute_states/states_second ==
  T_s : Inport
  T_c : Inport  Port=2
  T_t : Inport  Port=3
  wt_init1 : Inport  Port=4
  Enable : EnablePort  StatesWhenEnabling=reset
  Bus Selector3 : BusSelector  OutputSignals=tc3
  Constant26 : Constant  Value=0
  Gain{10,12,14..15} (4 alike) : Gain
  Gain11 : Gain  Gain=R2/R1
  Gain3 : Gain  Gain=R2*Rd
  Gain8 : Gain  Gain=1/It2
  Gain9 : Gain  Gain=R2
  Integrator1 : Integrator  InitialConditionSource=external  ShowStatePort=on
  Mux : Mux  Inputs=5
  Sum7 : Sum  Inputs=+-
  Terminator : Terminator
  states : Outport
  wt_dot : Outport  Port=2
  wcr_dot : Outport  Port=3
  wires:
  T_t/1 -> Sum7/1
  T_s/1 -> Gain3/1
  Gain3/1 -> Sum7/2
  T_c/1 -> Bus Selector3/1
  Sum7/1 -> Gain8/1
  Constant26/1 -> Mux/5  "wsr"
  Gain9/1 -> Mux/2  "wcr"
  Gain10/1 -> Mux/3  "wci"
  Gain11/1 -> Mux/4  "wsi"
  Gain12/1 -> Mux/1  "wt"
  Mux/1 -> states/1
  Integrator1/1 -> Gain12/1, Gain9/1, Gain10/1, Gain11/1
  Integrator1/State -> [wt_second], [wcr_second]
  wt_init1/1 -> Integrator1/2
  Gain8/1 -> Integrator1/1, Gain14/1, Gain15/1  "wt_dot"
  Gain14/1 -> wt_dot/1  "wt_dot"
  Gain15/1 -> wcr_dot/1  "wcr_dot"
  Bus Selector3/1 -> Terminator/1  "<tc3>"

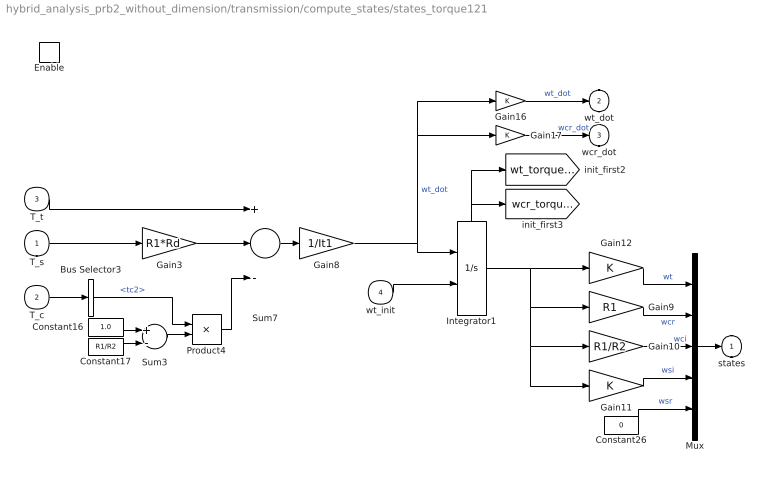
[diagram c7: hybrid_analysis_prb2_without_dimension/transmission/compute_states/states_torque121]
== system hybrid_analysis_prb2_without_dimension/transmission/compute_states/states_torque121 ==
  T_s : Inport
  T_c : Inport  Port=2
  T_t : Inport  Port=3
  wt_init : Inport  Port=4
  Enable : EnablePort  StatesWhenEnabling=reset
  Bus Selector3 : BusSelector  OutputSignals=tc2
  Constant16 : Constant  Value=1.0
  Constant17 : Constant  Value=R1/R2
  Constant26 : Constant  Value=0
  Gain10 : Gain  Gain=R1/R2
  Gain{11..12,16..17} (4 alike) : Gain
  Gain3 : Gain  Gain=R1*Rd
  Gain8 : Gain  Gain=1/It1
  Gain9 : Gain  Gain=R1
  Integrator1 : Integrator  InitialConditionSource=external  ShowStatePort=on
  Mux : Mux  Inputs=5
  Product4 : Product
  Sum3 : Sum  Inputs=+-
  Sum7 : Sum  Inputs=+--
  states : Outport
  wt_dot : Outport  Port=2
  wcr_dot : Outport  Port=3
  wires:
  T_t/1 -> Sum7/1
  T_s/1 -> Gain3/1
  Gain3/1 -> Sum7/2
  T_c/1 -> Bus Selector3/1
  Constant16/1 -> Sum3/1
  Constant17/1 -> Sum3/2
  Bus Selector3/1 -> Product4/1  "<tc2>"
  Product4/1 -> Sum7/3
  Sum7/1 -> Gain8/1
  Sum3/1 -> Product4/2
  wt_init/1 -> Integrator1/2
  Gain8/1 -> Integrator1/1, Gain17/1, Gain16/1  "wt_dot"
  Integrator1/State -> [wt_torque121], [wcr_torque121]
  Integrator1/1 -> Gain12/1, Gain9/1, Gain10/1, Gain11/1
  Gain9/1 -> Mux/2  "wcr"
  Gain11/1 -> Mux/4  "wsi"
  Gain10/1 -> Mux/3  "wci"
  Constant26/1 -> Mux/5  "wsr"
  Gain12/1 -> Mux/1  "wt"
  Mux/1 -> states/1
  Gain16/1 -> wt_dot/1  "wt_dot"
  Gain17/1 -> wcr_dot/1  "wcr_dot"

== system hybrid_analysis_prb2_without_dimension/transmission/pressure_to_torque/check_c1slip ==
  note: If fabs(C1slip) < 0.5 set it equal to 0.0
  In1 : Inport
  Abs : Abs
  Constant : Constant  Value=0.5
  Constant1 : Constant  Value=0
  Relational Operator : RelationalOperator  Operator=<
  Switch : Switch  Threshold=0.5
  Out1 : Outport
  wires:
  Constant/1 -> Relational Operator/2
  Switch/1 -> Out1/1  "c1slip"
  Relational Operator/1 -> Switch/2
  Abs/1 -> Relational Operator/1
  Constant1/1 -> Switch/1
  In1/1 -> Abs/1, Switch/3

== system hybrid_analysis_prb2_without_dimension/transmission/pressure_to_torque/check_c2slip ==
  note: If fabs(C2slip) < 0.5 set it equal to 0.0
  In1 : Inport
  Abs : Abs
  Constant : Constant  Value=0.5
  Constant1 : Constant  Value=0
  Relational Operator : RelationalOperator  Operator=<
  Switch : Switch  Threshold=0.5
  Out1 : Outport
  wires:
  Constant/1 -> Relational Operator/2
  Switch/1 -> Out1/1  "c2slip"
  Relational Operator/1 -> Switch/2
  Abs/1 -> Relational Operator/1
  Constant1/1 -> Switch/1
  In1/1 -> Abs/1, Switch/3

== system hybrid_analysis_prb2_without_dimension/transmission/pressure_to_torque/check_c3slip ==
  note: If fabs(C3slip) < 1.0 set it equal to 0.0
  In1 : Inport
  Abs : Abs
  Constant : Constant  Value=1.0
  Constant1 : Constant  Value=0
  Relational Operator : RelationalOperator  Operator=<
  Switch : Switch  Threshold=0.5
  Out1 : Outport
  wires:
  Constant/1 -> Relational Operator/2
  Switch/1 -> Out1/1  "c3slip"
  Relational Operator/1 -> Switch/2
  Abs/1 -> Relational Operator/1
  Constant1/1 -> Switch/1
  In1/1 -> Abs/1, Switch/3

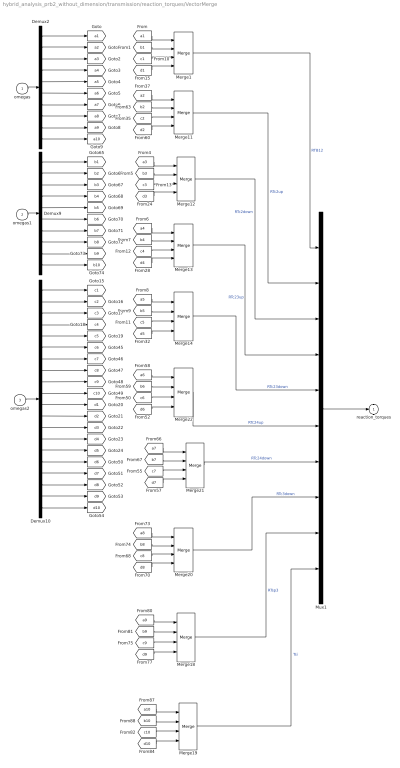
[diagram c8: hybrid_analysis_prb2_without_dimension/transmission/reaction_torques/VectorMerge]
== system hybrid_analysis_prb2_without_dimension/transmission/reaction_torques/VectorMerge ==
  omegas : Inport
  omegas1 : Inport  Port=2
  omegas2 : Inport  Port=3
  Demux10 : Demux  Outputs=20
  Demux2 : Demux  Outputs=10
  Demux9 : Demux  Outputs=10
  Merge{1,11..14,18..22} (10 alike) : Merge  Inputs=4
  Mux1 : Mux  Inputs=10
  reaction_torques : Outport  InitialOutput=[0,0,0,0,0,0,0,0,0,0]
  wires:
  omegas/1 -> Demux2/1
  Demux2/5 -> [a5]
  Demux2/4 -> [a4]
  Demux2/3 -> [a3]
  Demux2/2 -> [a2]
  Demux2/1 -> [a1]
  Demux2/7 -> [a7]
  Demux2/6 -> [a6]
  [a1] -> Merge1/1
  [b1] -> Merge1/2
  [c1] -> Merge1/3
  [d1] -> Merge1/4
  Demux2/8 -> [a8]
  Demux2/10 -> [a10]
  Demux2/9 -> [a9]
  omegas1/1 -> Demux9/1
  Demux9/5 -> [b5]
  Demux9/4 -> [b4]
  Demux9/3 -> [b3]
  Demux9/2 -> [b2]
  Demux9/1 -> [b1]
  Demux9/7 -> [b7]
  Demux9/6 -> [b6]
  Demux9/8 -> [b8]
  Demux9/10 -> [b10]
  Demux9/9 -> [b9]
  [a2] -> Merge11/1
  [b2] -> Merge11/2
  [c2] -> Merge11/3
  [d2] -> Merge11/4
  omegas2/1 -> Demux10/1
  Demux10/5 -> [c5]
  Demux10/4 -> [c4]
  Demux10/3 -> [c3]
  Demux10/2 -> [c2]
  Demux10/1 -> [c1]
  Demux10/7 -> [c7]
  Demux10/6 -> [c6]
  Demux10/8 -> [c8]
  Demux10/10 -> [c10]
  Demux10/9 -> [c9]
  Demux10/15 -> [d5]
  Demux10/14 -> [d4]
  Demux10/13 -> [d3]
  Demux10/12 -> [d2]
  Demux10/11 -> [d1]
  Demux10/17 -> [d7]
  Demux10/16 -> [d6]
  Demux10/18 -> [d8]
  Demux10/20 -> [d10]
  Demux10/19 -> [d9]
  [a3] -> Merge12/1
  [b3] -> Merge12/2
  [c3] -> Merge12/3
  [d3] -> Merge12/4
  [a4] -> Merge13/1
  [b4] -> Merge13/2
  [c4] -> Merge13/3
  [d4] -> Merge13/4
  [a5] -> Merge14/1
  [b5] -> Merge14/2
  [c5] -> Merge14/3
  [d5] -> Merge14/4
  [a6] -> Merge22/1
  [b6] -> Merge22/2
  [c6] -> Merge22/3
  [d6] -> Merge22/4
  [a7] -> Merge21/1
  [b7] -> Merge21/2
  [c7] -> Merge21/3
  [d7] -> Merge21/4
  [a8] -> Merge20/1
  [b8] -> Merge20/2
  [c8] -> Merge20/3
  [d8] -> Merge20/4
  [a9] -> Merge18/1
  [b9] -> Merge18/2
  [c9] -> Merge18/3
  [d9] -> Merge18/4
  Merge14/1 -> Mux1/5  "RTc23down"
  Merge1/1 -> Mux1/1  "RTB12"
  Merge19/1 -> Mux1/10  "Tsi"
  Merge18/1 -> Mux1/9  "RTsp3"
  Merge11/1 -> Mux1/2  "RTc2up"
  Merge20/1 -> Mux1/8  "RTc3down"
  Merge21/1 -> Mux1/7  "RTc24down"
  Merge13/1 -> Mux1/4  "RTc23up"
  Merge12/1 -> Mux1/3  "RTc2down"
  Mux1/1 -> reaction_torques/1
  Merge22/1 -> Mux1/6  "RTc24up"
  [a10] -> Merge19/1
  [b10] -> Merge19/2
  [c10] -> Merge19/3
  [d10] -> Merge19/4

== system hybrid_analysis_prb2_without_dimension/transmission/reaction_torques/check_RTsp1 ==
  note: If |RTsp1| < 1 set it equal to 0.0
  note: Change around rtsp1 to see effects on model.....code does something strange here. JSS
  In1 : Inport
  In2 : Inport  Port=2
  Abs : Abs
  Constant : Constant  Value=1.0
  Constant1 : Constant  Value=0
  Relational Operator : RelationalOperator  Operator=<
  Switch : Switch  Threshold=0.5
  Terminator2 : Terminator
  Out1 : Outport
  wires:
  Constant/1 -> Relational Operator/2
  Relational Operator/1 -> Switch/2
  Constant1/1 -> Switch/1
  In2/1 -> Terminator2/1
  Switch/1 -> Out1/1  "RTsp1"
  In1/1 -> Abs/1
  Abs/1 -> Relational Operator/1, Switch/3

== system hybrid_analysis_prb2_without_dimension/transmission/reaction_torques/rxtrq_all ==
  T_c : Inport
  T_s : Inport  Port=2
  T_t : Inport  Port=3
  omega_dots : Inport  Port=4
  Bus Selector : BusSelector  OutputSignals=tc2
  Bus Selector1 : BusSelector  OutputSignals=wt_dot,wcr_dot
  Gain2 : Gain  Gain=R1*Rd
  Gain3 : Gain  Gain=It
  Gain4 : Gain  Gain=R1/R2
  Gain5 : Gain  Gain=Isi12/R1
  Sum : Sum  Inputs=+--
  Sum1 : Sum  Inputs=+-+
  RTc1up : Outport  InitialOutput=[0,0,0,0,0,0,0,0,0,0]
  RTsp1 : Outport  Port=2  InitialOutput=[0,0,0,0,0,0,0,0,0,0]
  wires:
  T_t/1 -> Sum/1
  Sum/1 -> RTc1up/1  "RTc1up"
  Gain3/1 -> Sum/3
  Bus Selector/1 -> Sum/2, Gain4/1  "<tc2>"
  Bus Selector1/1 -> Gain3/1  "<wt_dot>"
  omega_dots/1 -> Bus Selector1/1
  T_c/1 -> Bus Selector/1
  Bus Selector1/2 -> Gain5/1  "<wcr_dot>"
  Gain5/1 -> Sum1/1
  Gain4/1 -> Sum1/2
  Sum1/1 -> RTsp1/1  "RTsp1"
  Gain2/1 -> Sum1/3
  T_s/1 -> Gain2/1

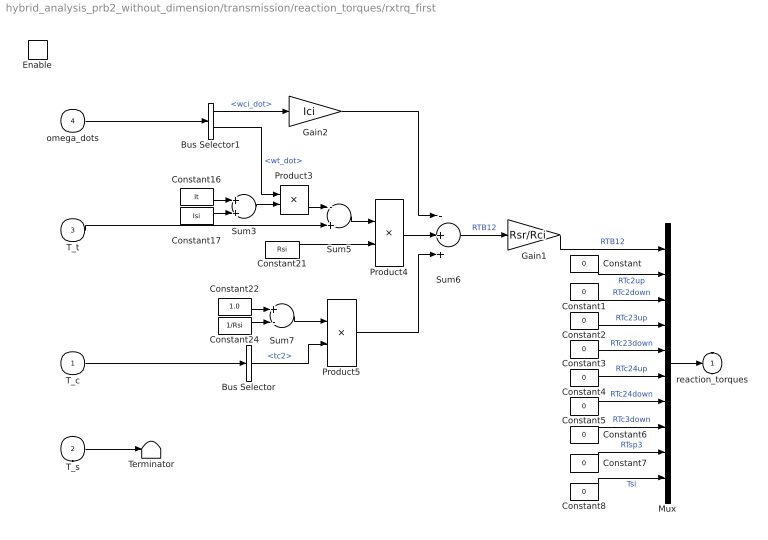
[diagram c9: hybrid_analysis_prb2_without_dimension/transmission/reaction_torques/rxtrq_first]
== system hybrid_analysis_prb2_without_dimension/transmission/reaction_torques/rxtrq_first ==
  T_c : Inport
  T_s : Inport  Port=2
  T_t : Inport  Port=3
  omega_dots : Inport  Port=4
  Enable : EnablePort  StatesWhenEnabling=reset
  Bus Selector : BusSelector  OutputSignals=tc2
  Bus Selector1 : BusSelector  OutputSignals=wci_dot,wt_dot
  Constant{,1..8} (9 alike) : Constant  Value=0
  Constant16 : Constant  Value=It
  Constant17 : Constant  Value=Isi
  Constant21 : Constant  Value=Rsi
  Constant22 : Constant  Value=1.0
  Constant24 : Constant  Value=1/Rsi
  Gain1 : Gain  Gain=Rsr/Rci
  Gain2 : Gain  Gain=Ici
  Mux : Mux  Inputs=10
  Product3 : Product
  Product4 : Product  Inputs=*/
  Product5 : Product
  Sum3 : Sum
  Sum5 : Sum  Inputs=-+
  Sum6 : Sum  Inputs=-++
  Sum7 : Sum  Inputs=+-
  Terminator : Terminator
  reaction_torques : Outport
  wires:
  Constant16/1 -> Sum3/1
  Constant17/1 -> Sum3/2
  Sum3/1 -> Product3/2
  Product3/1 -> Sum5/1
  T_t/1 -> Sum5/2
  omega_dots/1 -> Bus Selector1/1
  Bus Selector1/2 -> Product3/1  "<wt_dot>"
  Sum5/1 -> Product4/1
  Constant21/1 -> Product4/2
  Bus Selector1/1 -> Gain2/1  "<wci_dot>"
  Product4/1 -> Sum6/2
  Gain2/1 -> Sum6/1
  T_c/1 -> Bus Selector/1
  Bus Selector/1 -> Product5/2  "<tc2>"
  Constant22/1 -> Sum7/1
  Sum7/1 -> Product5/1
  Product5/1 -> Sum6/3
  Sum6/1 -> Gain1/1  "RTB12"
  Constant/1 -> Mux/2  "RTc2up"
  Constant1/1 -> Mux/3  "RTc2down"
  Constant2/1 -> Mux/4  "RTc23up"
  Constant3/1 -> Mux/5  "RTc23down"
  Mux/1 -> reaction_torques/1
  Constant8/1 -> Mux/10  "Tsi"
  Constant7/1 -> Mux/9  "RTsp3"
  Constant6/1 -> Mux/8  "RTc3down"
  Constant5/1 -> Mux/7  "RTc24down"
  Constant4/1 -> Mux/6  "RTc24up"
  T_s/1 -> Terminator/1
  Gain1/1 -> Mux/1  "RTB12"
  Constant24/1 -> Sum7/2

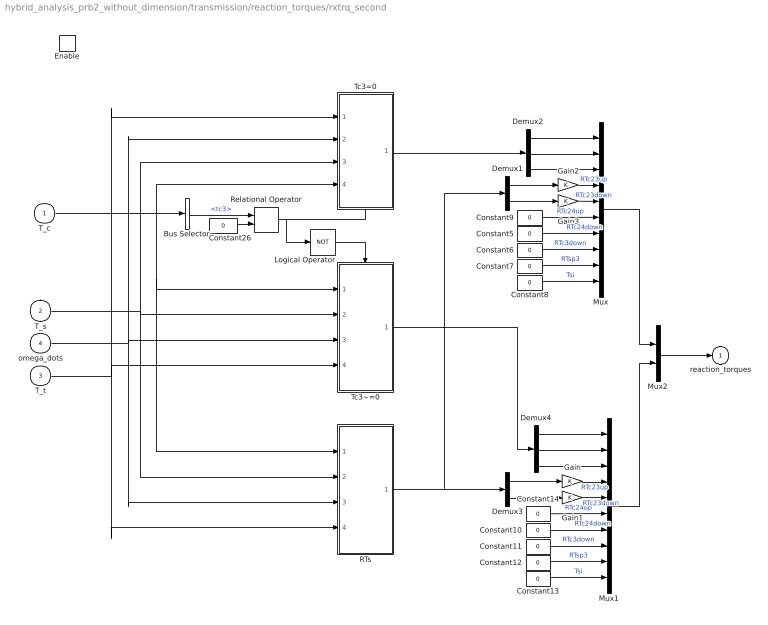
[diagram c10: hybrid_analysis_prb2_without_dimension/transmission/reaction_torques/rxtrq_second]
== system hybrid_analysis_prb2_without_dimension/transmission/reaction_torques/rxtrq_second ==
  T_c : Inport
  T_s : Inport  Port=2
  T_t : Inport  Port=3
  omega_dots : Inport  Port=4
  Enable : EnablePort  StatesWhenEnabling=reset
  Bus Selector : BusSelector  OutputSignals=tc3
  Constant{5..14,26} (11 alike) : Constant  Value=0
  Demux1 : Demux  Outputs=2
  Demux2 : Demux  Outputs=3
  Demux3 : Demux  Outputs=2
  Demux4 : Demux  Outputs=3
  Gain{,1..3} (4 alike) : Gain
  Logical Operator : Logic  Operator=NOT
  Mux : Mux  Inputs=10
  Mux1 : Mux  Inputs=10
  Mux2 : Mux  Inputs=2
  RTs : Subsystem
  Relational Operator : RelationalOperator  Operator===
  Tc3=0 : Subsystem  TreatAsAtomicUnit=on
  Tc3~=0 : Subsystem  TreatAsAtomicUnit=on
  reaction_torques : Outport
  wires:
  Bus Selector/1 -> Relational Operator/1  "<tc3>"
  Constant26/1 -> Relational Operator/2
  Relational Operator/1 -> Tc3=0/Enable, Logical Operator/1
  Logical Operator/1 -> Tc3~=0/Enable
  T_c/1 -> Bus Selector/1, Tc3=0/4(T_c), Tc3~=0/1(T_c), RTs/1(T_c)
  T_s/1 -> Tc3=0/3(T_s), Tc3~=0/2(T_s), RTs/2(T_s)
  T_t/1 -> Tc3=0/1(T_t), Tc3~=0/4(T_t), RTs/4(T_t)
  omega_dots/1 -> Tc3=0/2(omega_dots), Tc3~=0/3(omega_dots), RTs/3(omega_dots)
  Constant8/1 -> Mux/10  "Tsi"
  Constant7/1 -> Mux/9  "RTsp3"
  Constant6/1 -> Mux/8  "RTc3down"
  Constant5/1 -> Mux/7  "RTc24down"
  Constant9/1 -> Mux/6  "RTc24up"
  Demux2/1 -> Mux/1
  Demux2/3 -> Mux/3
  Demux2/2 -> Mux/2
  Tc3=0/1(RTs) -> Demux2/1
  Constant13/1 -> Mux1/10  "Tsi"
  Constant12/1 -> Mux1/9  "RTsp3"
  Constant11/1 -> Mux1/8  "RTc3down"
  Constant10/1 -> Mux1/7  "RTc24down"
  Constant14/1 -> Mux1/6  "RTc24up"
  Demux4/1 -> Mux1/1
  Demux4/3 -> Mux1/3
  Demux4/2 -> Mux1/2
  RTs/1(RTs) -> Demux3/1, Demux1/1
  Tc3~=0/1(RTs) -> Demux4/1
  Mux2/1 -> reaction_torques/1
  Mux/1 -> Mux2/1
  Mux1/1 -> Mux2/2
  Demux3/1 -> Gain/1
  Gain/1 -> Mux1/4  "RTc23up"
  Demux3/2 -> Gain1/1
  Gain1/1 -> Mux1/5  "RTc23down"
  Demux1/1 -> Gain2/1
  Gain2/1 -> Mux/4  "RTc23up"
  Demux1/2 -> Gain3/1
  Gain3/1 -> Mux/5  "RTc23down"

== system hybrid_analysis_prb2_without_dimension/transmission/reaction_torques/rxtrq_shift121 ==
  T_c : Inport
  T_s : Inport  Port=2
  T_t : Inport  Port=3
  omega_dots : Inport  Port=4
  Enable : EnablePort  StatesWhenEnabling=reset
  Bus Selector : BusSelector  OutputSignals=tc2
  Bus Selector1 : BusSelector  OutputSignals=wci_dot,wsi_dot,wt_dot
  Constant{2..8} (7 alike) : Constant  Value=0
  Gain1 : Gain  Gain=Rsr/Rci
  Gain2 : Gain  Gain=It
  Gain3 : Gain  Gain=R2*Rd
  Gain4 : Gain  Gain=Ici12
  Gain5 : Gain  Gain=Ici
  Gain6 : Gain  Gain=Isi/Rsi
  Mux : Mux  Inputs=10
  Sum4 : Sum
  Sum5 : Sum  Inputs=-+
  Sum6 : Sum  Inputs=+--
  reaction_torques : Outport
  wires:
  Bus Selector/1 -> Sum6/1  "<tc2>"
  omega_dots/1 -> Bus Selector1/1
  Bus Selector1/2 -> Gain6/1  "<wsi_dot>"
  Gain6/1 -> Sum6/3
  Gain5/1 -> Sum6/2
  Sum6/1 -> Gain1/1
  Constant4/1 -> Mux/6  "RTc24up"
  Constant5/1 -> Mux/7  "RTc24down"
  Constant6/1 -> Mux/8  "RTc3down"
  Constant7/1 -> Mux/9  "RTsp3"
  Constant8/1 -> Mux/10  "Tsi"
  Mux/1 -> reaction_torques/1
  Constant3/1 -> Mux/5  "RTc23down"
  Constant2/1 -> Mux/4  "RTc23up"
  T_t/1 -> Sum5/2
  Bus Selector1/3 -> Gain2/1  "<wt_dot>"
  Gain2/1 -> Sum5/1
  Sum5/1 -> Mux/2  "RTc2up"
  Gain1/1 -> Mux/1  "RTB12"
  Bus Selector1/1 -> Gain5/1, Gain4/1  "<wci_dot>"
  Gain4/1 -> Sum4/1
  Sum4/1 -> Mux/3  "RTc2down"
  Gain3/1 -> Sum4/2
  T_s/1 -> Gain3/1
  T_c/1 -> Bus Selector/1

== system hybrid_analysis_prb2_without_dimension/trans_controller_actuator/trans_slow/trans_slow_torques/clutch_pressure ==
  ngear1 : Inport
  Gain : Gain  Gain=Pc1max
  Gain1 : Gain  Gain=Pc2max
  Gain2 : Gain  Gain=Pc3max
  c1_table : Lookup  InputValues=pres_index  Table=c1_table.y
  c2_table : Lookup  InputValues=pres_index  Table=c2_table.y
  c3_table : Lookup  InputValues=pres_index  Table=c3_table.y
  Pc5 : Outport  InitialOutput=0
  Pc6 : Outport  Port=2  InitialOutput=0
  Pc7 : Outport  Port=3  InitialOutput=0
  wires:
  Gain2/1 -> Pc7/1  "pc3"
  Gain1/1 -> Pc6/1  "pc2"
  Gain/1 -> Pc5/1  "pc1"
  c3_table/1 -> Gain2/1  "c3_on_off"
  c2_table/1 -> Gain1/1  "c2_on_off"
  c1_table/1 -> Gain/1  "c1_on_off"
  ngear1/1 -> c2_table/1, c3_table/1, c1_table/1
